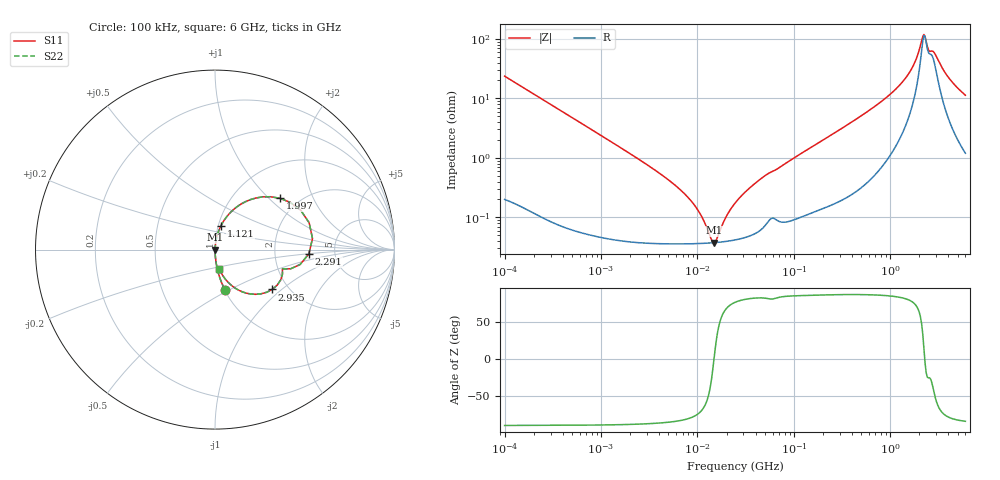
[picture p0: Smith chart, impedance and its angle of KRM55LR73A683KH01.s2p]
!Murata Part Number: KRM55LR73A683KH01
!These Parameters are Measured in Series Mode Connection
!Data Generated on Jan 08, 2026
!  o--ll--o
!Port1  Port2
!  o------o
!Operation Temp=25[degC], DC Bias Voltage=0[V]
!Freq. Start=100[kHz] Stop=6[GHz] 401[Steps]
# Hz S RI R 50
!Freq.(Hz) S11(Real) S11(Imag) S21(Real) S21(Imag) S12(Real) S12(Imag) S22(Real) S22(Imag)
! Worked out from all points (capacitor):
!   401 points, 100 kHz to 6 GHz, reference 50 ohm
!   read as one part in series: C = 67.3 nF near 105.7 kHz
!   lowest |Z| = 37.5 mohm at 14.93 MHz (marker M1)
!   series resonance near 14.85 MHz, so ESL is about 1.7 nH
!   S11 on the Smith chart (normalised r, x): 100 kHz: 1.00, -0.47; 1.121 GHz: 1.03, +0.28; 1.997 GHz: 1.61, +1.17; 2.291 GHz: 3.18, -0.21; 2.935 GHz: 1.65, -0.86; 6 GHz: 1.02, -0.22
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100000  0.0545 -0.2228  0.9455 0.2228  0.9455 0.2228  0.0545 -0.2228
631452  0.00196 -0.0376  0.998 0.0376  0.998 0.0376  0.00196 -0.0376
3987316  0.000391 -0.00556  0.9996 0.00556  0.9996 0.00556  0.000391 -0.00556
8853126  0.000362 -0.00174  0.9996 0.00174  0.9996 0.00174  0.000362 -0.00174
1.103214e7  0.000365 -0.00097  0.9996 0.00097  0.9996 0.00097  0.000365 -0.00097
1.413084e7  0.000372 -0.000159  0.9996 0.000159  0.9996 0.000159  0.000372 -0.000159
1.492997e7  0.000375 1.81e-05  0.9996 -1.81e-05  0.9996 -1.81e-05  0.000375 1.81e-05
1.577428e7  0.000378 0.000195  0.9996 -0.000195  0.9996 -0.000195  0.000378 0.000195
2.020496e7  0.000396 0.00101  0.9996 -0.00101  0.9996 -0.00101  0.000396 0.00101
2.517799e7  0.000423 0.00178  0.9996 -0.00178  0.9996 -0.00178  0.000423 0.00178
4.872031e7  0.000708 0.00479  0.9993 -0.00479  0.9993 -0.00479  0.000708 0.00479
1.546735e8  0.00142 0.0153  0.9986 -0.0153  0.9986 -0.0153  0.00142 0.0153
9.76689e8  0.0227 0.1098  0.9773 -0.1098  0.9773 -0.1098  0.0227 0.1098
1.120684e9  0.0329 0.1322  0.9671 -0.1322  0.9671 -0.1322  0.0329 0.1322
1.647094e9  0.13 0.2439  0.87 -0.2439  0.87 -0.2439  0.13 0.2439
1.996807e9  0.3612 0.2862  0.6388 -0.2862  0.6388 -0.2862  0.3612 0.2862
2.168564e9  0.5247 0.1495  0.4753 -0.1495  0.4753 -0.1495  0.5247 0.1495
2.2912e9  0.523 -0.024  0.477 0.024  0.477 0.024  0.523 -0.024
2.55767e9  0.376 -0.1065  0.624 0.1065  0.624 0.1065  0.376 -0.1065
2.934752e9  0.3188 -0.2219  0.6812 0.2219  0.6812 0.2219  0.3188 -0.2219
3.863894e9  0.0967 -0.2035  0.9033 0.2035  0.9033 0.2035  0.0967 -0.2035
6e9  0.0238 -0.1083  0.9762 0.1083  0.9762 0.1083  0.0238 -0.1083
